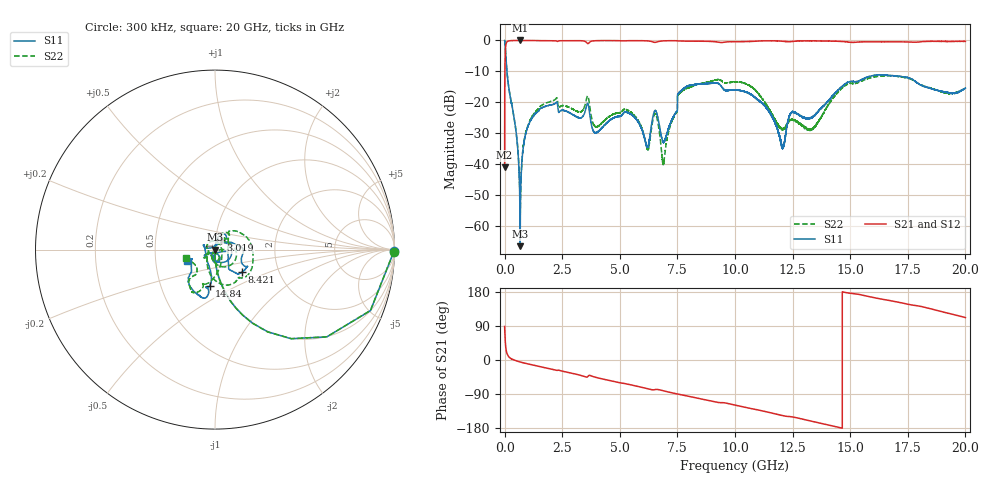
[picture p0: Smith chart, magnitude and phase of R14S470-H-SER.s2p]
!{R14S470}
!Johanson Technology Inc.
!www.johansontechnology.com
!Test Board Conditions:
!Substrate Type  RO4350B
!Substrate Thickness  20 mil
!Substrate Dk  3.66
!TL Type: GCPW
!TL Trace Width  36 mil
!TL Gap  12 mil
!Electrode orientation  Horizontal
!DUT TOPOLOGY	SERIES
!Mounting Pad LxW  26x36 mil
! Created Wed Nov 25 17:33:21 2020
! 2 Port Network Data from SP1.SP block
! freq  magS11  angS11  magS21  angS21  magS12  angS12  magS22  angS22
# khz S ma R 50
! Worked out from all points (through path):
!   20001 points, 300 kHz to 20 GHz, reference 50 ohm
!   highest |S21| = 0.00 dB at 669.3 MHz (marker M1); lowest = -41.1 dB at 300 kHz (marker M2)
!   group delay of S21, straight-line fit = 34.4 ps
!   lowest |S11| = -66.6 dB at 674.3 MHz (marker M3), VSWR 1.00, Z = 50 - j0.0187 ohm
!   |S11| at or under -10 dB: 99.82 MHz to end of sweep
!   |S22| runs from -54.8 to 0.0 dB; largest |S21 - S12| = 0.017
!   S11 on the Smith chart (normalised r, x): 300 kHz: open; 3.019 GHz: 1.06, +0.11; 8.421 GHz: 1.31, -0.34; 14.84 GHz: 0.87, -0.37; 20 GHz: 0.72, -0.10
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300  0.9968 -0.6  0.008817 88.6  0.008846 89.2  0.9949 -0.8
118300  0.2689 -75.1  0.9615 14.6  0.9618 14.6  0.27 -75.1
669300  0.001155 -117.2  0.9997 -5.2  0.9985 -5.1  0.002107 -39.3
674300  0.0004688 -156.5  0.9989 -5.2  0.9991 -5.2  0.002099 -22.6
916300  0.03106 84.1  0.9986 -9.0  0.9987 -9.0  0.03163 74.9
1306300  0.06315 78.5  0.995 -14.5  0.9958 -14.5  0.06764 70.7
3019300  0.06137 57.6  0.9903 -36.4  0.9911 -36.3  0.07516 48.5
3334300  0.05617 49.3  0.9884 -41.2  0.9885 -41.1  0.07084 38.1
5352300  0.06776 -151.6  0.9903 -63.9  0.9907 -63.9  0.0738 -148.2
6187300  0.01894 -105.9  0.9841 -75.3  0.985 -75.3  0.01771 -114.3
6667300  0.05298 -105.5  0.9575 -77.9  0.9582 -78.0  0.0439 -114.9
6904300  0.02255 -61.4  0.9851 -81.5  0.9853 -81.5  0.0103 -45.2
7600300  0.1471 -52.5  0.9813 -91.1  0.9819 -91.1  0.1399 47.9
8421300  0.1961 -39.5  0.9723 -101.4  0.9707 -101.3  0.1964 14.4
1.00003e7  0.1577 -2.3  0.9534 -119.0  0.9521 -119.0  0.2141 -60.8
1.13173e7  0.08544 29.3  0.9855 -136.0  0.9844 -136.1  0.09684 -115.7
1.20643e7  0.01823 112.1  0.9727 -146.6  0.973 -146.5  0.03666 -166.4
1.24503e7  0.067 160.5  0.9567 -149.8  0.9595 -149.8  0.05236 139.3
1.33343e7  0.05579 -150.6  0.9841 -161.7  0.9843 -161.7  0.03683 6.8
1.48393e7  0.205 -98.6  0.949 177.6  0.9492 177.4  0.1922 -102.5
1.66673e7  0.2698 -108.1  0.9513 157.4  0.9447 157.2  0.2702 -118.0
2e7  0.1691 -157.1  0.9653 111.9  0.9639 112.3  0.1704 -164.0
